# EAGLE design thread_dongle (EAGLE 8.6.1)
AUTHOR: Joshua Adkins, Neal Jackson; REV: A; TITLE: Thread Dongle
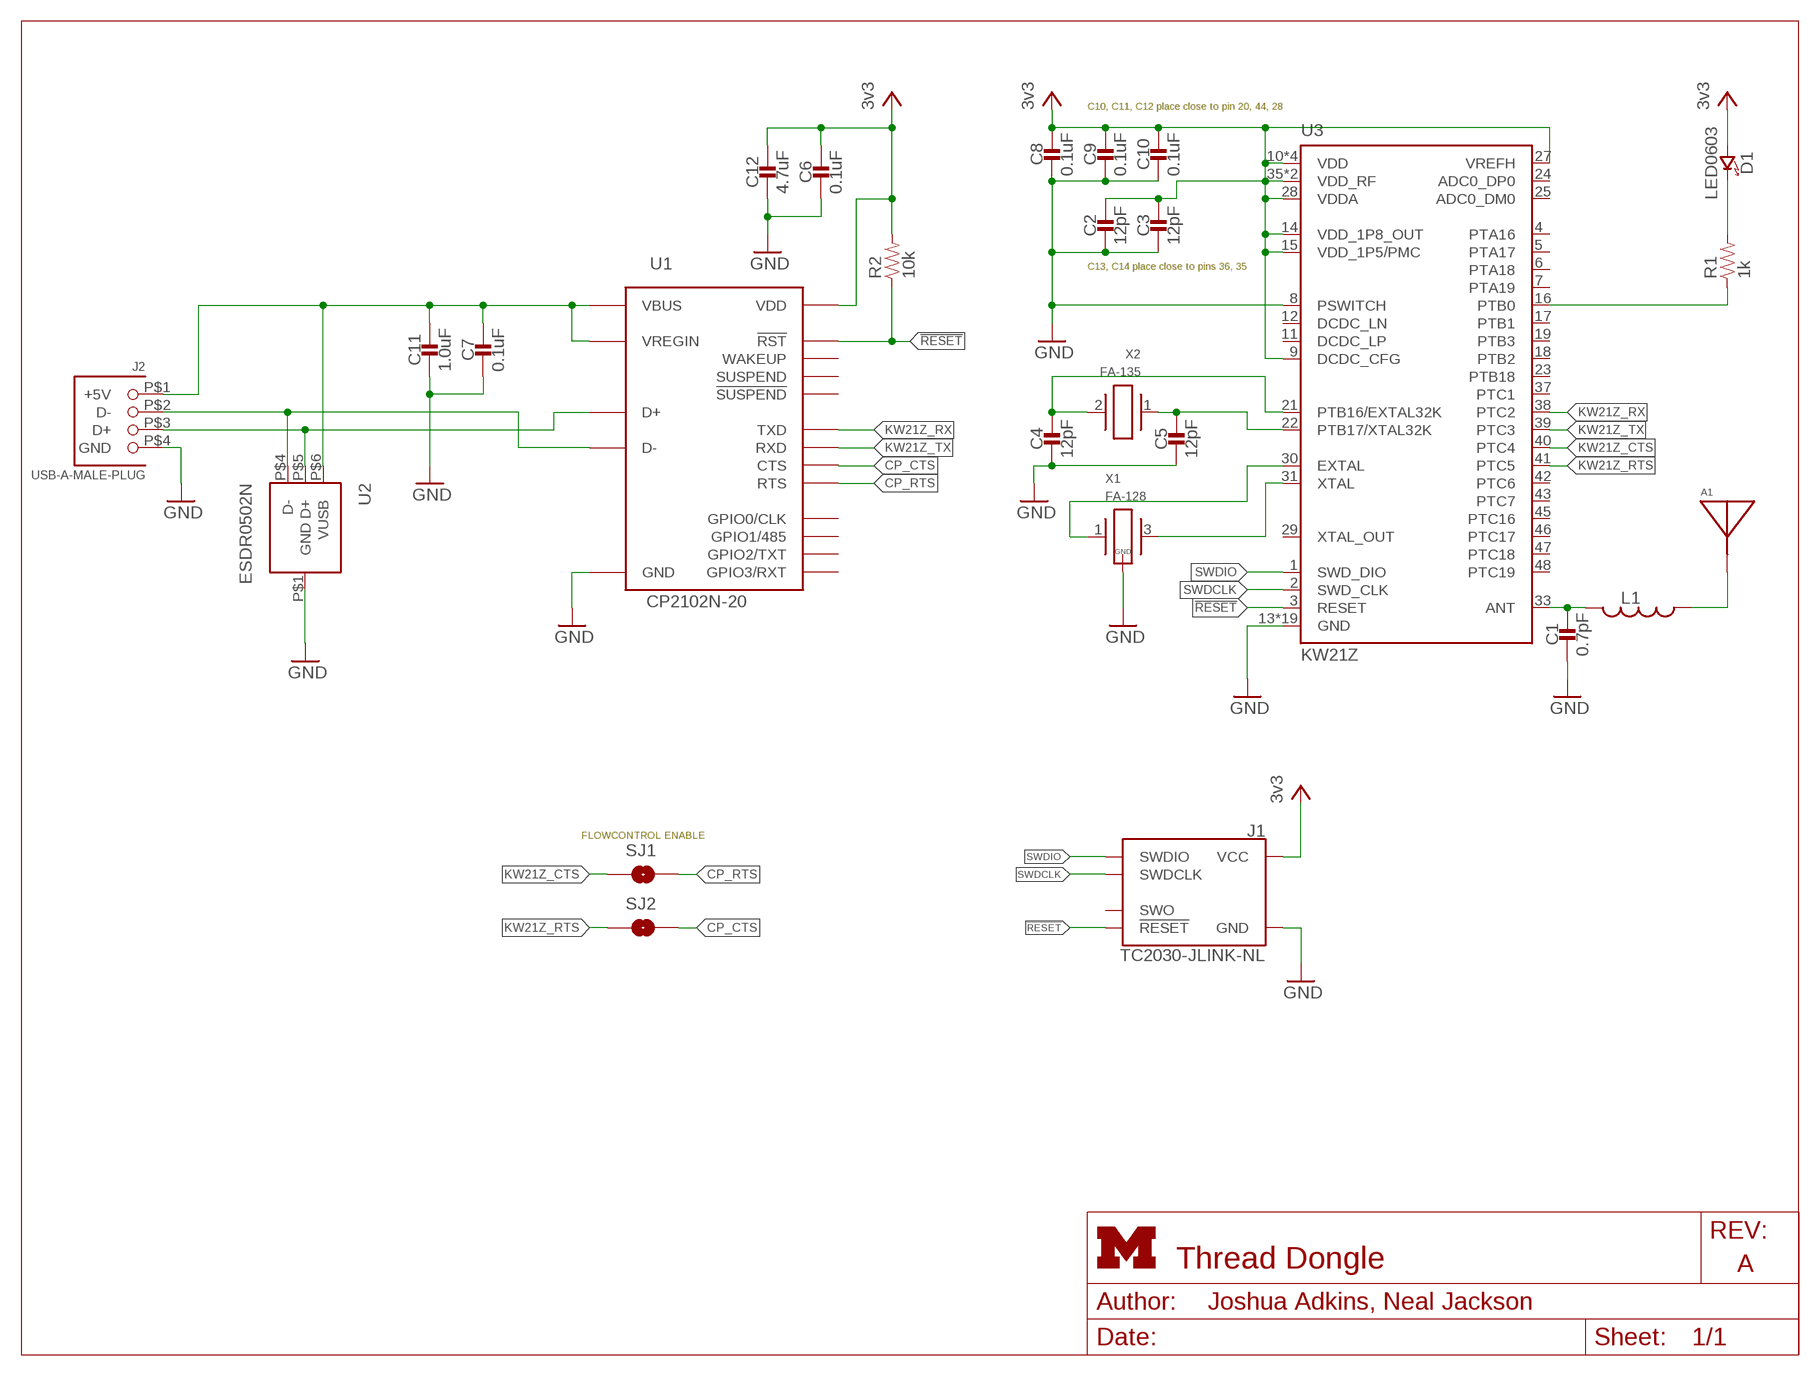
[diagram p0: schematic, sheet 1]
FRAME1 (LETTER_L_UMICH): HEIGHT: 8.5in; WIDTH: 11in

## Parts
A1  AH212M  [AH212M]
C1  0.7pF  CAPACITOR0402_CAP  [0402_CAP]
C2  12pF  CAPACITOR0402_CAP  [0402_CAP]
C3  12pF  CAPACITOR0402_CAP  [0402_CAP]
C4  12pF  CAPACITOR0402_CAP  [0402_CAP]
C5  12pF  CAPACITOR0402_CAP  [0402_CAP]
C6  0.1uF  CAPACITOR0402_CAP  [0402_CAP]
C7  0.1uF  CAPACITOR0402_CAP  [0402_CAP]
C8  0.1uF  CAPACITOR0402_CAP  [0402_CAP]
C9  0.1uF  CAPACITOR0402_CAP  [0402_CAP]
C10  0.1uF  CAPACITOR0402_CAP  [0402_CAP]
C11  1.0uF  CAPACITOR0402_CAP  [0402_CAP]
C12  4.7uF  CAPACITOR0402_CAP  [0402_CAP]
D1  LED0603  [LED-0603]
J1  TC2030-JLINK-NL  [TC2030-IDC-NL]
J2  USB-A-MALE-PLUG  [USB_A_MALE_PLUG_CUI_UP2-AH]
L1  INDUCTOR0402  [0402_CAP]
R1  1k  RESISTOR0402_RES  [0402_RES]
R2  10k  RESISTOR0402_RES  [0402_RES]
SJ1  SOLDERJUMPERNC  [SJ_2S_SMALL]
SJ2  SOLDERJUMPERNC  [SJ_2S_SMALL]
U1  CP2102N-20  [QFN-20-3MM]
U2  ESDR0502N  [UDFN-6]
U3  KW21Z  [LAMINATE-QFN-48-7MM]
X1  FA-128  [FA-128]
X2  FA-135  [FC-135]

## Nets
5V: C7.1 C11.1 J2.P$1(+5V) U1.7(VREGIN) U1.8(VBUS) U2.P$6(VUSB)
!RESET: J1.3(!RESET) R2.1 U1.9(!RST) U3.3(RESET)
CP_CTS: SJ2.2 U1.15(CTS)
CP_RTS: SJ1.2 U1.16(RTS)
D+: J2.P$3(D+) U1.4(D+) U2.P$5(D+)
D-: J2.P$2(D-) U1.5(D-) U2.P$4(D-)
GND: C1.2 C2.2 C3.2 C4.2 C5.2 C6.2 C7.2 C8.2 C9.2 C10.2 C11.2 C12.2 J1.5(GND) J2.P$4(GND) U1.3(GND) U1.12(GND) U1.P$1(GND) U2.P$1(GND) U3.8(PSWITCH) U3.13(GND) U3.26(GND) U3.34(GND) U3.49(GND) U3.50(GND) U3.51(GND) U3.52(GND) U3.53(GND) U3.54(GND) U3.55(GND) U3.56(GND) U3.57(GND) U3.58(GND) U3.59(GND) U3.60(GND) U3.61(GND) U3.62(GND) U3.63(GND) U3.64(GND) X1.2(GND) X1.4(GND)
KW21Z_CTS: SJ1.1 U3.40(PTC4)
KW21Z_RTS: SJ2.1 U3.41(PTC5)
KW21Z_RX: U1.18(TXD) U3.38(PTC2)
KW21Z_TX: U1.17(RXD) U3.39(PTC3)
N$1: C4.1 U3.21(PTB16/EXTAL32K) X2.2
N$2: C5.1 U3.22(PTB17/XTAL32K) X2.1
N$3: U3.31(XTAL) X1.3
N$7: D1.C(CATHODE) R1.2
N$8: R1.1 U3.16(PTB0)
N$12: U3.30(EXTAL) X1.1
N$13: C1.1 L1.2 U3.33(ANT)
N$16: A1.P1(ANTENNA) L1.1
SWDCLK: J1.4(SWDCLK) U3.2(SWD_CLK)
SWDIO: J1.2(SWDIO) U3.1(SWD_DIO)
VCC: C2.1 C3.1 C6.1 C8.1 C9.1 C10.1 C12.1 D1.A(ANODE) J1.1(VCC) R2.2 U1.6(VDD) U3.9(DCDC_CFG) U3.10(VDD) U3.14(VDD_1P8_OUT) U3.15(VDD_1P5/PMC) U3.20(VDD) U3.27(VREFH) U3.28(VDDA) U3.32(VDD) U3.35(VDD_RF) U3.36(VDD_RF) U3.44(VDD) ; supply symbol labelled 3v3
Unconnected: J1.6(SWO) U1.1(GPIO1/485) U1.2(GPIO0/CLK) U1.11(!SUSPEND) U1.13(WAKEUP) U1.14(SUSPEND) U1.19(GPIO3/RXT) U1.20(GPIO2/TXT) U3.4(PTA16) U3.5(PTA17) U3.6(PTA18) U3.7(PTA19) U3.11(DCDC_LP) U3.12(DCDC_LN) U3.17(PTB1) U3.18(PTB2) U3.19(PTB3) U3.23(PTB18) U3.24(ADC0_DP0) U3.25(ADC0_DM0) U3.29(XTAL_OUT) U3.37(PTC1) U3.42(PTC6) U3.43(PTC7) U3.45(PTC16) U3.46(PTC17) U3.47(PTC18) U3.48(PTC19)

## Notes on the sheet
- C10, C11, C12 place close to pin 20, 44, 28
- C13, C14 place close to pins 36, 35
- FLOWCONTROL ENABLE

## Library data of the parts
A1 = chips:AH212M: Small 2.4Ghz chip antenna; DIGIKEY: 587-2725-1-ND; MPN: AH212M245001-T
C1 = passives:CAPACITOR: SMD Capacitor; DIGIKEY: 490-6267-1-ND; MPN: GRM1555C1HR70BA01D
C2-C5 = passives:CAPACITOR: SMD Capacitor; DIGIKEY: 490-5924-1-ND; MPN: GRM1555C1H120JA01D
C6-C10 = passives:CAPACITOR: SMD Capacitor; DIGIKEY: 587-1227-1-ND; MPN: LMK105BJ104KV-F
C11 = passives:CAPACITOR: SMD Capacitor; DIGIKEY: 490-10018-1-ND; MPN: GRM155R61E105MA12D
C12 = passives:CAPACITOR: SMD Capacitor; DIGIKEY: 490-5915-1-ND; MPN: GRM155R60J475ME47D
D1 = leds:LED: LED; DIGIKEY: 160-1837-6-ND; MPN: LTST-C194TBKT
J1 = connector:TC2030-JLINK
J2 = connector:USB-A-MALE-PLUG: USB A Male plug connector; DIGIKEY: 102-3996-ND; MANUFACTURER: CUI; MPN: UP2-AH-1-TH
L1 = passives:INDUCTOR: A very specific inductor; DIGIKEY: 490-6573-1-ND; MPN: LQG15HS5N1S02D
R1 = passives:RESISTOR: Resistor; DIGIKEY: 311-1.0KJRCT-ND; MPN: RC0402JR-071KL
R2 = passives:RESISTOR: Resistor; DIGIKEY: 311-10KJRCT-ND; MPN: RC0402JR-0710KL
SJ1 SJ2 = headers:SOLDERJUMPER: Solder Jumper
U1 = chips:CP2102N-20: A cheap, simple USB to UART adapter; DIGIKEY: 336-3692-ND; MANUFACTURER: SiLabs; MPN: CP2102N-A01-GQFN20
U2 = chips:ESDR0502N; DIGIKEY: ESDR0502NMUTBGOSCT-ND; MPN: ESDR0502NMUTBG
U3 = chips:KW21Z: NXP KW21Z Cortex M0+ 802.15.4; DIGIKEY: MKW21Z256VHT4-ND; MPN: MKW21Z256VHT4
X1 = crystals:FA-128: Epson MHz RANGE CRYSTAL UNIT ULTRA MINIATURE SIZE LOW PROFILE SMD http://www.digikey.com/product-search/en?FV=ffec63d1; DIGIKEY: SER4079CT-ND; MPN: FA-128 32.0000MF20X-K5
X2 = crystals:FA-135: Epson kHz RANGE CRYSTAL UNIT; DIGIKEY: SER4086CT-ND; MPN: FC-135 32.7680KA-AG3

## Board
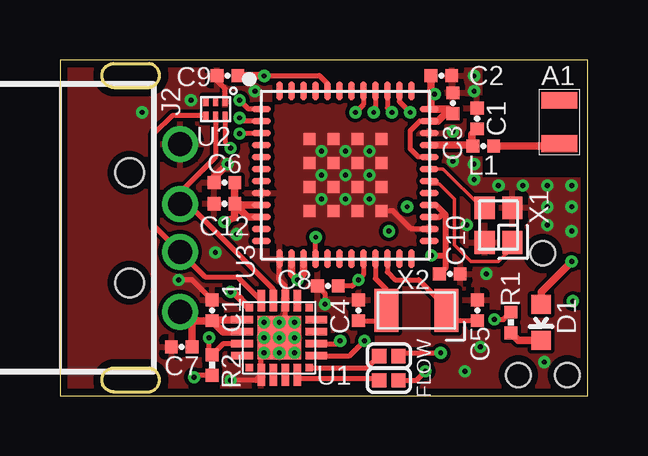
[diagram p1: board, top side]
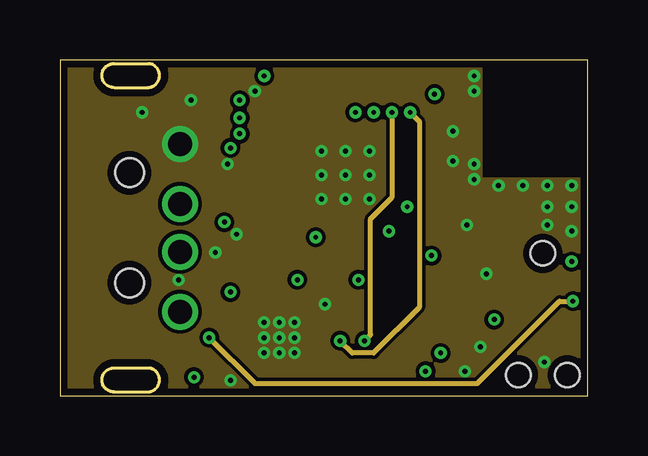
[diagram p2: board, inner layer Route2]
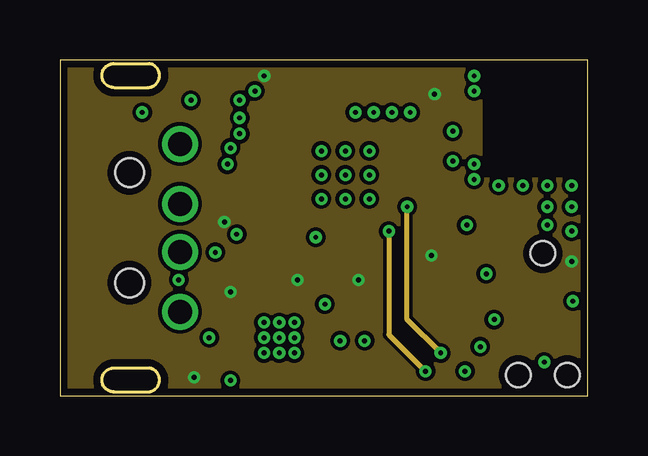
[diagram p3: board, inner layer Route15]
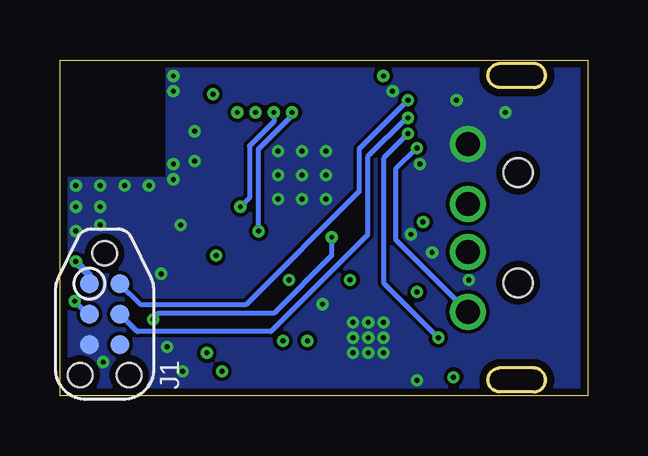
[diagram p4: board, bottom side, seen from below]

Size 22 x 14 mm. Coordinates in mm from the lower left corner, seen from the top.
Outline: 0,0 22,0 22,14 0,14 0,0
Copper layers (1+2*15+16): Top 0.0178mm / dielectric 59mil / Route2 0.0356mm / dielectric 0.1499mm / Route15 0.0356mm / dielectric 0.2007mm / Bottom 0.0178mm
Design rules "quickturn_co_kr_1oz_4lyr *": minimum track width 6mil, minimum drill 8mil, track to track 6mil, track to pad 6mil, pad to pad 6mil, via to via 6mil, smd to smd 6mil, copper to edge 12mil, drill to drill 12mil, minimum pad ring 8mil, minimum via ring 6mil, stop-mask expansion 3mil, vias tented up to drill 50mil, thermal gap 10mil

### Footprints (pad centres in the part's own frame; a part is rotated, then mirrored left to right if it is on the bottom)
AH212M = smd 1.5 x 0.7: P1 0,0.35; P2 0,2.15
0402_CAP = smd 0.536 x 0.546: 1 -0.433,0; 2 0.433,0
LED-0603 = smd 0.8 x 0.8: A 0,-0.75; C 0,0.75
TC2030-IDC-NL = smd 0.787 x 0.787: 1 -1.27,-0.635; 2 -1.27,0.635; 3 0,-0.635; 4 0,0.635; 5 1.27,-0.635; 6 1.27,0.635 | hole 1.016: -2.54,0; 2.54,1.016; 2.54,-1.016
USB_A_MALE_PLUG_CUI_UP2-AH = drill 1: P$1 3.5,5; P$2 1,5; P$3 -1,5; P$4 -3.5,5 | hole 1.2: -2.3,2.9; 2.3,2.9
0402_RES = smd 0.536 x 0.546: 1 -0.433,0; 2 0.433,0
SJ_2S_SMALL = smd 0.6 x 0.6: 1 -0.4,0; 2 0.4,0
QFN-20-3MM = smd 0.3 x 0.3: 1 -1.25,1.25; 6 -1.25,-1.25; 11 1.25,-1.25; 16 1.25,1.25 | smd 0.9 x 0.3: 2 -1.55,0.75; 3 -1.55,0.25; 4 -1.55,-0.25; 5 -1.55,-0.75; 12 1.55,-0.75; 13 1.55,-0.25; 14 1.55,0.25; 15 1.55,0.75 | smd 0.3 x 0.9: 7 -0.75,-1.55; 8 -0.25,-1.55; 9 0.25,-1.55; 10 0.75,-1.55; 17 0.75,1.55; 18 0.25,1.55; 19 -0.25,1.55; 20 -0.75,1.55 | smd 1.8 x 1.8: P$1 0,0
UDFN-6 = smd 0.42 x 0.22: P$1 -0.325,0.4; P$2 -0.325,0; P$3 -0.325,-0.4; P$4 0.325,-0.4; P$5 0.325,0; P$6 0.325,0.4
LAMINATE-QFN-48-7MM = smd 0.8 x 0.28: 1 -3.5,2.75; 2 -3.5,2.25; 3 -3.5,1.75; 4 -3.5,1.25; 5 -3.5,0.75; 6 -3.5,0.25; 7 -3.5,-0.25; 8 -3.5,-0.75; 9 -3.5,-1.25; 10 -3.5,-1.75; 11 -3.5,-2.25; 12 -3.5,-2.75; 25 3.5,-2.75; 26 3.5,-2.25; 27 3.5,-1.75; 28 3.5,-1.25; 29 3.5,-0.75; 30 3.5,-0.25; 31 3.5,0.25; 32 3.5,0.75; 33 3.5,1.25; 34 3.5,1.75; 35 3.5,2.25; 36 3.5,2.75 | smd 0.28 x 0.8: 13 -2.75,-3.5; 14 -2.25,-3.5; 15 -1.75,-3.5; 16 -1.25,-3.5; 17 -0.75,-3.5; 18 -0.25,-3.5; 19 0.25,-3.5; 20 0.75,-3.5; 21 1.25,-3.5; 22 1.75,-3.5; 23 2.25,-3.5; 24 2.75,-3.5; 37 2.75,3.5; 38 2.25,3.5; 39 1.75,3.5; 40 1.25,3.5; 41 0.75,3.5; 42 0.25,3.5; 43 -0.25,3.5; 44 -0.75,3.5; 45 -1.25,3.5; 46 -1.75,3.5; 47 -2.25,3.5; 48 -2.75,3.5 | smd 0.5 x 0.5: 49 -1.5,1.5; 50 -0.5,1.5; 51 0.5,1.5; 52 1.5,1.5; 53 -1.5,0.5; 54 -0.5,0.5; 55 0.5,0.5; 56 1.5,0.5; 57 -1.5,-0.5; 58 -0.5,-0.5; 59 0.5,-0.5; 60 1.5,-0.5; 61 -1.5,-1.5; 62 -0.5,-1.5; 63 0.5,-1.5; 64 1.5,-1.5
FA-128 = smd 0.95 x 0.85: 1 -0.725,-0.575; 2 0.725,-0.575; 3 0.725,0.575; 4 -0.725,0.575
FC-135 = smd 1 x 1.8: 1 -1.25,0; 2 1.25,0

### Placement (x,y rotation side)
A1  20.82,10.16 0 top
C1  17.39,11.56 90 top
C2  15.9,13.34 0 top
C3  16.38,12.19 90 top
C4  12.45,3.56 90 top
C5  17.4,3.56 90 top
C6  6.86,8.89 180 top
C7  5.08,2.03 180 top
C8  11.17,4.57 180 top
C9  6.99,13.34 180 top
C10  16.26,5.08 0 top
C11  6.35,3.56 90 top
C12  6.86,8 180 top
D1  20.07,3.05 180 top
J1  20.14,3.4 270 bottom
J2  0,7 270 top
L1  17.65,10.41 180 top
R1  18.8,3.05 270 top
R2  6.35,1.27 270 top
SJ1  13.72,1.65 180 top
SJ2  13.72,0.64 180 top
U1  9.14,2.41 270 top
U2  6.49,11.96 270 top
U3  11.9,9.2 0 top
X1  18.29,7.11 90 top
X2  14.86,3.56 180 top

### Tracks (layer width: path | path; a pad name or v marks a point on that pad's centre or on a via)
5V  (via drill 0.2)
  Top 0.203: v7.11,10.33 6.89,10.55 U2.P$6
  Top 0.305: J2.P$1 5.38,3.12 5.59,3.12 | 5.59,3.12 C11.1 | U1.8 6.81,2.66 C11.1 | U1.7 6.39,3.16 C11.1 | C7.1 5.51,3.05 5.59,3.12
  Bottom 0.203: J2.P$1 8,6.5 8,9.44 v7.11,10.33
!RESET  (via drill 0.2)
  Top 0.203: U1.9 6.81,2.16 R2.1 6.22,1.83 v6.22,2.41 | U3.3 8.37,10.92 v7.49,10.92
  Route2 0.203: v6.22,2.41 8.13,0.51 17.4,0.51 20.83,3.94 v21.39,3.94
  Bottom 0.203: v6.22,2.41 8.51,4.7 8.51,9.91 v7.49,10.92 | J1.3 20.92,3.4 20.92,3.47 v21.39,3.94
CP_CTS
  Top 0.203: U1.15 10.03,0.72 13.23,0.72 SJ2.2
CP_RTS
  Top 0.203: U1.16 12.81,1.16 13.3,1.65 SJ1.2
D+
  Top 0.203: U1.4 8.89,4.44 5.33,8 J2.P$3 5,8.47 6.49,9.96 U2.P$5
D-
  Top 0.203: 7.91,4.45 U1.5 7.4,4.95 6.05,4.95 J2.P$2 3.94,7.06 3.94,10.92 4.7,11.68 6.03,11.68 U2.P$4
GND  (via drill 0.2)
  Top 0.203: C11.2 5.51,4.83 v4.95,4.83 | C8.2 11.05,4.26 v11.05,3.81 | U3.13 9.14,4.83 9.39,4.58 U1.3 9.39,3.3 v9.14,3.05 | U2.P$1 6.89,12.8 6.55,13.13 C9.2 | v8.51,1.78 8.39,1.66 U1.12 8.17,0.64 v7.11,0.64 | U3.26 14.64,6.95 13.89,7.7 U3.64
  Top 0.305: C6.2 6.42,9.09 v6.99,9.65
  other vias: 17.53,2.03 16.89,1.02 20.19,1.4 17.27,12.7 17.27,13.34 17.27,9.65 17.27,9.02 18.29,8.76 19.3,8.76 20.32,8.76 21.34,8.76 10.9,8.2 11.9,8.2 12.9,8.2 12.9,9.2 11.9,9.2 10.9,9.2 10.9,10.2 11.9,10.2 12.9,10.2 17.78,5.08 21.34,7.87 20.32,7.87 21.34,6.86 20.32,7.11 16.38,9.78 16.38,11.02 6.48,5.97 5.46,12.32 3.43,11.81 8.13,12.7 9.14,2.41 8.51,2.41 8.51,3.05 9.78,3.05 9.78,2.41 9.78,1.78 9.14,1.78 16.97,7.11 7.37,6.73
  pour Top (isolate 0.102): -1.52,0 -1.52,14 17.51,14 17.51,9 22,9 21.92,0
  pour Route2 (isolate 0.102, no thermals): -1.02,0 -1.02,14.1 17.51,14 17.51,9 22,9 21.92,0
  pour Bottom (isolate 0.102, no thermals): 0,0 0,14.1 17.51,14 17.51,9 22,9 21.92,0
  pour Top (rank 2, no thermals): 9.91,11.18 13.97,11.18 13.97,7.24 9.91,7.24
KW21Z_CTS  (via drill 0.2)
  Top 0.203: 14.23,1.78 SJ1.1 14.24,1.78 v15.88,1.78 | U3.40 13.15,11.88 v13.08,11.81
  Route15 0.203: v15.88,1.78 14.48,3.17 v14.48,7.87
  Bottom 0.203: v13.08,11.81 13.08,11.43 14.1,10.41 14.1,8.26 v14.48,7.87
KW21Z_RTS  (via drill 0.2)
  Top 0.203: SJ2.1 14.86,0.64 v15.24,1.02 | U3.41 12.65,12.14 v12.32,11.81
  Route15 0.203: v13.72,6.86 13.72,2.54 v15.24,1.02
  Bottom 0.203: v13.72,6.86 13.72,10.29 12.32,11.68 v12.32,11.81
KW21Z_RX  (via drill 0.2)
  Top 0.203: U1.18 11.56,2.16 v11.68,2.29 | U3.38 14.15,12.27 v14.61,11.81
  Route2 0.203: v11.68,2.29 12.19,1.78 13.08,1.78 14.99,3.68 14.99,11.43 v14.61,11.81
KW21Z_TX  (via drill 0.2)
  Top 0.152: U3.39 13.67,12.67
  Top 0.203: U1.17 12.08,1.66 v12.7,2.29 | U3.39 13.65,12 v13.84,11.81
  Route2 0.203: v13.84,11.81 13.84,8.26 12.95,7.37 12.95,2.54 v12.7,2.29
N$1
  Top 0.203: U3.21 13.15,4.88 13.61,4.42 X2.2 13.18,3.12 C4.1
N$2
  Top 0.203: U3.22 13.65,5.15 13.97,4.83 14.97,4.83 16.11,3.68 X2.1 16.54,3.12 C5.1
N$3
  Top 0.152: U3.31 15.97,9.45 17.59,7.84 X1.3
N$7
  Top 0.305: R1.2 19.11,2.3 D1.C
N$8  (via drill 0.2)
  Top 0.203: U3.16 10.65,6.59 v10.67,6.6 | R1.1 18.49,3.17 v18.11,3.17
  Bottom 0.203: v10.67,6.6 10.67,5.84 13.08,3.43 17.91,3.43 18.11,3.23 v18.11,3.17
N$12
  Top 0.152: U3.30 15.53,8.82 15.81,8.82 16.44,8.19 16.44,6.29 17.14,5.59 18.29,5.59 18.86,6.16 X1.1
N$13
  Top 0.203: U3.33 15.47,10.41
  Top 0.305: U3.33 17.18,10.45 | 17.18,10.45 L1.2 | C1.1 17.18,10.91 17.18,10.45
N$16
  Top 0.305: L1.1 20.73,10.41 A1.P1
SWDCLK  (via drill 0.2)
  Top 0.203: U3.2 7.62,11.45 v7.49,11.58
  Bottom 0.203: J1.4 18.77,2.67 13.21,2.67 9.17,6.71 9.17,9.96 7.55,11.58 v7.49,11.58
SWDIO  (via drill 0.2)
  Top 0.203: U3.1 7.86,11.95 v7.49,12.32
  Bottom 0.203: J1.2 18.64,3.81 14.22,3.81 9.53,8.51 9.53,10.29 v7.49,12.32
VCC  (via drill 0.2)
  Top 0.203: R2.2 5.66,0.84 v5.59,0.76 | U3.20 12.65,5.03 v12.45,4.83 12.19,4.57 C8.1 11.56,4.52 | U3.32 14.94,9.95 14.61,10.29 14.61,11.05 15.01,11.45 U3.35 | U3.44 11.15,13.02 10.81,13.35 8.54,13.35 v8.52,13.33
  Top 0.254: U3.27 15.83,7.45 16,7.62 | U3.28 15.67,7.95 16,7.62 | 16.08,5.84 16.08,7.54 16,7.62 | 16.08,5.84 16.08,5.33 C10.1 | v15.49,5.84 16.08,5.84
  Top 0.305: C2.1 15.47,12.45 | 15.47,12.45 15.47,12.02 U3.36 16.19,11.95 16.23,11.91 | v15.62,12.57 15.59,12.57 15.47,12.45 | D1.A 20.07,4.32 v21.34,5.59 | U3.9 7.34,7.95 C12.1 | U3.10 7.83,7.45 C12.1 | U1.6 7.24,4.32 v7.11,4.32 | C12.1 7.29,7.42 v6.86,7.24 | C12.1 C6.1 | C9.1 v8.51,13.34 v8.52,13.33 | 16.23,11.91 C3.1 | U3.35 15.77,11.45 16.23,11.91 | U3.14 9.65,5.08 v9.91,4.83 10.15,5.07 U3.15
  Bottom 0.305: v21.34,5.59 20.77,5.02 J1.1
  pour Route15 (isolate 0.102, no thermals): -0.51,0 -0.51,14.1 17.51,14 17.51,9 22,9 21.92,0

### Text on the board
tPlace: FLOW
